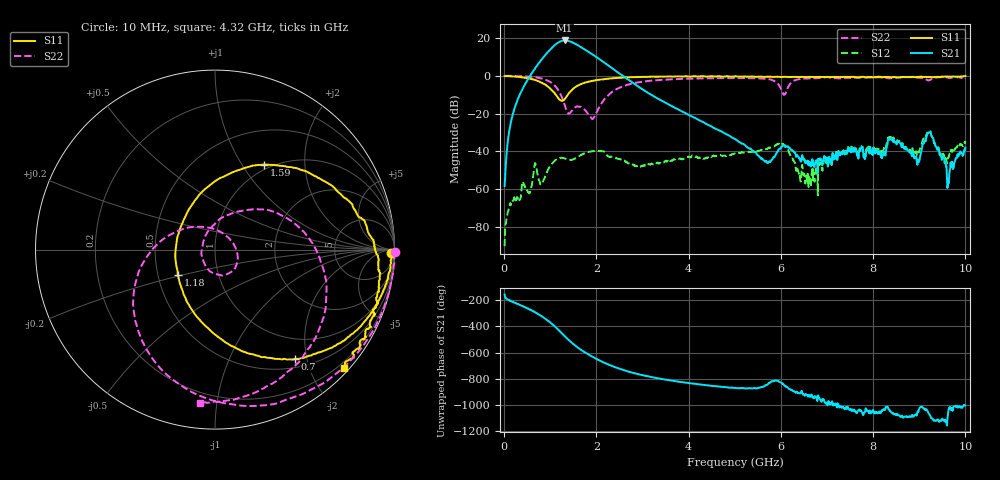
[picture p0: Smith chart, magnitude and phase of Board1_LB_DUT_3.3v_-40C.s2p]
! Created Tue May 27 16:02:18 2025
# hz S ma R 50
! 2 Port Network Data from SP1.SP block
! freq  magS11  angS11  magS21  angS21  magS12  angS12  magS22  angS22
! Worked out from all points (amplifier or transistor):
!   1000 points, 10 MHz to 10 GHz, reference 50 ohm
!   highest |S21| = 18.8 dB at 1.31 GHz (marker M1)
!   |S21| within 3 dB of that: 1.072 GHz to 1.631 GHz (558.8 MHz wide, 41.4 % of centre)
!   unconditionally stable (mu >= 1): 19.5 MHz to 24.23 MHz; 56.83 MHz to 64.27 MHz; 87.59 MHz to end of sweep
!   at 1.67 GHz: K = 6.76, MAG = 17.3 dB, |S12| = -41.9 dB
!   at 5.01 GHz: K = 30.65, MAG = -14.1 dB, |S12| = -41.3 dB
!   at 10 GHz: K = 9.95, MAG = -14.7 dB, |S12| = -34.5 dB
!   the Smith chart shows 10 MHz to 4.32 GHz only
!   S11 on the Smith chart (normalised r, x): 10 MHz: 58, -49; 700 MHz: 0.64, -1.79; 1.18 GHz: 0.63, -0.19; 1.59 GHz: 0.93, +1.26; 4.32 GHz: 0.09, -2.57
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1e7  0.9802 -1.0  0.00119 -157.1  3.022e-05 129.2  1.005 -0.8
2.1e8  0.9638 -14.5  0.119 143.5  0.0005364 82.0  0.9957 -18.9
7e8  0.7535 -53.9  1.771 62.2  0.003532 60.5  0.9116 -72.1
9.4e8  0.5298 -82.1  4.195 6.6  0.003017 114.5  0.7504 -110.4
1.07e9  0.3773 -107.2  6.128 -30.8  0.005187 98.5  0.5932 -138.6
1.18e9  0.2512 -145.7  7.765 -67.1  0.006504 78.8  0.405 -169.9
1.25e9  0.2177 174.8  8.463 -91.7  0.006647 67.3  0.2746 164.1
1.31e9  0.239 137.4  8.698 -113.0  0.006469 60.4  0.1743 133.2
1.44e9  0.3875 88.5  8.113 -156.4  0.005908 57.6  0.1083 17.5
1.59e9  0.547 59.9  6.582 160.9  0.007014 58.6  0.1543 -51.2
1.68e9  0.6139 48.6  5.651 138.7  0.008077 53.9  0.144 -78.7
1.91e9  0.7358 29.6  3.738 89.7  0.01 31.0  0.07158 175.8
2.13e9  0.8051 17.0  2.451 49.8  0.009983 6.0  0.2033 70.4
2.55e9  0.8959 -0.8  1.042 -8.7  0.005908 -12.3  0.5141 9.4
3.34e9  0.9518 -21.8  0.2459 -75.7  0.004701 10.6  0.7709 -50.4
4.32e9  0.9756 -42.6  0.059 -126.5  0.006285 0.0  0.856 -95.6
5.01e9  0.9755 -56.1  0.02079 -148.7  0.008637 -8.8  0.8754 -119.6
6.67e9  0.9379 -88.2  0.005461 159.7  0.002893 168.6  0.8617 -150.4
8.34e9  0.9266 -133.6  0.01993 49.5  0.02268 54.7  0.8596 167.4
9.23e9  0.9313 -157.7  0.03147 5.0  0.03362 12.0  0.7764 161.6
9.63e9  0.9506 -168.2  0.001507 33.3  0.006994 53.5  0.8925 153.1
1e10  0.9925 -179.7  0.01247 77.5  0.01873 68.0  0.8449 144.5
